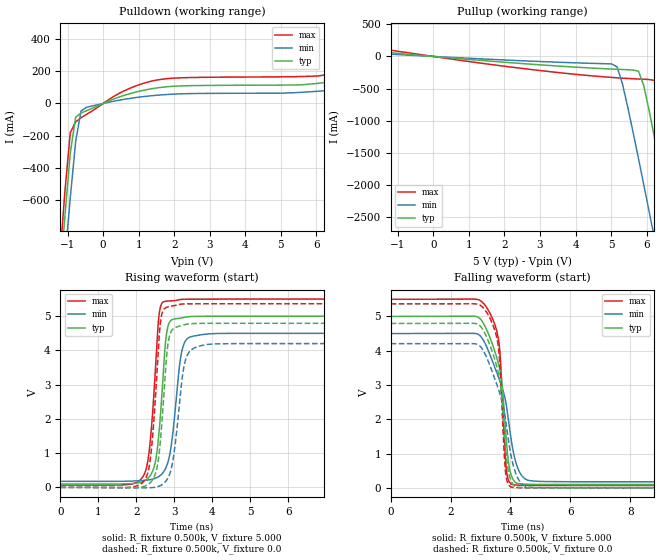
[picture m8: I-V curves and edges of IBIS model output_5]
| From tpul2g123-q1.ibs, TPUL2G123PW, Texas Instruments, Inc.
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|   Model output_5
[Model] output_5
Model_type Output
Polarity   Non-Inverting
Enable   Active-High
Vmeas = 5v
Cref = 15pf
C_comp   1.934pF   1.732pF   2.140pF
[Temperature Range]   27.000   0.125k   -40.000
[Voltage Range]   5.000V   4.500V   5.500V
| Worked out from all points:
|   slope of the pulldown table from 0 to 0.75 V, typ, clamps not added: 12.3 ohm
|   slope of the pullup table from 0 to 0.75 V, typ, clamps not added: 21.5 ohm
|   rising waveform, R_fixture 0.500k, V_fixture 5.000: 20-80 % time 203ps typ, 254ps min, 206ps max; typ from 0.099 V to 5 V
|   rising waveform, R_fixture 0.500k, V_fixture 0.0: 20-80 % time 201ps typ, 258ps min, 202ps max; typ from 0 V to 4.8 V
|   falling waveform, R_fixture 0.500k, V_fixture 5.000: 20-80 % time 428ps typ, 673ps min, 231ps max; typ from 5 V to 0.099 V
|   falling waveform, R_fixture 0.500k, V_fixture 0.0: 20-80 % time 416ps typ, 643ps min, 226ps max; typ from 4.8 V to 0 V
[Pulldown]
|Voltage   I(typ)   I(min)   I(max)
-5V       -9.726A    -9.168A    -10.4A
-1.225V   -1.125A    -1.38A     -993.9mA
-1.074V   -700.8mA   -975.1mA   -545.1mA
-923mV    -306.7mA   -585.8mA   -181.3mA
-772mV    -84.87mA   -235.5mA   -114mA
-621mV    -59.47mA   -46.04mA   -89.2mA
-470mV    -45.05mA   -24.16mA   -68.14mA
436mV     39.09mA    19.86mA    61mA
1.342V    90.91mA    47.73mA    138mA
6.476V    136.5mA    84.04mA    186.4mA
8.288V    210.7mA    130.5mA    294.9mA
10V       325.8mA    125.2mA    469.7mA
[Pullup]
|Voltage   I(typ)   I(min)   I(max)
-5V       242.5mA    149.7mA    413.5mA
5.017V    -195.7mA   -115.9mA   -325.4mA
5.168V    -199.4mA   -161.1mA   -331.2mA
5.319V    -202.8mA   -425.4mA   -336.7mA
5.772V    -229.4mA   -1.589A    -350.3mA
6.074V    -851.5mA   -2.418A    -358.6mA
6.225V    -1.273A    -2.837A    -371.2mA
6.376V    -1.706A    -3.251A    -395.5mA
6.678V    -2.587A    -3.93A     -1.117A
7.131V    -3.923A    -4.787A    -2.506A
7.282V    -4.348A    -5.07A     -2.976A
10V       -9.866A    -10.17A    -9.592A
[Ramp]
| variable   typ   min   max
dV/dt_r   2.878/0.201n   2.524/0.257n   3.220/0.202n
dV/dt_f   2.941/0.428n   2.594/0.673n   3.259/0.231n
R_load = 0.500k
[Rising Waveform]
R_fixture= 0.500k
V_fixture= 5.000
V_fixture_min= 4.500
V_fixture_max= 5.500
|time   V(typ)   V(min)   V(max)
0s        98.59mV    177.2mV    68.56mV
2.177ns   173.1mV    200.6mV    318.9mV
2.367ns   350.7mV    226.3mV    1.364V
2.518ns   859.3mV    274.7mV    3.756V
2.619ns   1.905V     340.1mV    5.199V
2.811ns   4.602V     669.7mV    5.442V
2.924ns   4.89V      1.274V     5.451V
3.178ns   4.948V     3.873V     5.491V
4.144ns   4.999V     4.496V     5.499V
50ns      5V         4.5V       5.5V
[Rising Waveform]
R_fixture= 0.500k
V_fixture= 0.0
V_fixture_min= 0.0
V_fixture_max= 0.0
|time   V(typ)   V(min)   V(max)
0s        1.155uV    795.9nV    1.76uV
2.221ns   38.05mV    -13.51mV   217.8mV
2.39ns    165.6mV    -7.992mV   1.051V
2.656ns   1.669V     65.75mV    4.984V
2.847ns   4.294V     310.6mV    5.278V
2.99ns    4.649V     987.2mV    5.308V
3.196ns   4.73V      3.104V     5.356V
3.415ns   4.781V     3.989V     5.363V
4.025ns   4.793V     4.191V     5.364V
50ns      4.796V     4.206V     5.366V
[Falling Waveform]
R_fixture= 0.500k
V_fixture= 5.000
V_fixture_min= 4.500
V_fixture_max= 5.500
|time   V(typ)   V(min)   V(max)
0s        5V         4.5V       5.5V
2.789ns   5.005V     4.506V     5.504V
3.192ns   4.638V     4.14V      5.279V
3.605ns   3.598V     3.218V     4.305V
3.72ns    3.003V     2.93V      2.824V
3.867ns   1.337V     2.382V     513.7mV
4.122ns   200.8mV    942.1mV    90.43mV
4.392ns   113.4mV    341.2mV    75.03mV
5ns       99.89mV    186.5mV    69.12mV
50ns      98.59mV    177.2mV    68.56mV
[Falling Waveform]
R_fixture= 0.500k
V_fixture= 0.0
V_fixture_min= 0.0
V_fixture_max= 0.0
|time   V(typ)   V(min)   V(max)
0s        4.796V     4.206V     5.366V
2.824ns   4.794V     4.202V     5.366V
3.184ns   4.438V     3.845V     5.147V
3.584ns   3.396V     2.916V     4.183V
3.688ns   2.853V     2.63V      2.889V
3.829ns   1.257V     2.037V     523.2mV
4.065ns   129.6mV    756.3mV    15.66mV
4.385ns   8.163mV    113.8mV    3.854mV
4.925ns   652.9uV    5.661mV    414.6uV
50ns      467.8nV    1.998uV    117.3nV
